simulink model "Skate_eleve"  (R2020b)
settings: Solver=VariableStepAuto  StartTime=0.0  StopTime=10.0  RelTol=1e-3
libraries: fl_lib x8, nesl_utility x4, ee_lib x2, sdl_lib x2

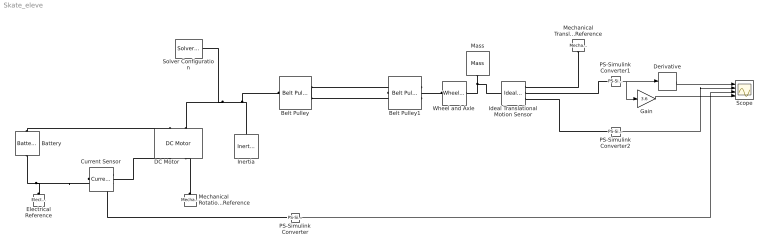
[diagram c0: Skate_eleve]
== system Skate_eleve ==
  Battery : ee_lib/Sources/Battery  Vnom=36 V  prm_dir=1  R1_dis=2 Ohm  R1_ch=2 Ohm  R1=2 Ohm  prm_AH=1  AH=50 hr*A  V1=11.5 V  AH1=25 hr*A  prm_R2=1  R2=2000 Ohm  prm_dyn=1  Rp1=0.005 Ohm  tau1=30 s  Rp2=0.005 Ohm  tau2=30 s  Rp3=0.005 Ohm  tau3=30 s  Rp4=0.005 Ohm  tau4=30 s  Rp5=0.005 Ohm  tau5=30 s  prm_fade=1  N_fade=100  AH_fade=45 hr*A  R1_fade=2.02 Ohm  R1_ch_fade=2.02 Ohm  V1_fade=10.35 V  i_specify=off  i_priority=None  i=0 A  i_nominal_specify=off  i_nominal_unit=A  i_nominal_value=1  v_specify=off  v_priority=None  v=0 V  v_nominal_specify=off  v_nominal_unit=V  v_nominal_value=1  charge_specify=off  charge_priority=High  charge=50 hr*A  charge_nominal_specify=off  charge_nominal_unit=hr*A  charge_nominal_value=1  num_cycles_specify=off  num_cycles_priority=High  num_cycles=0  num_cycles_nominal_specify=off  num_cycles_nominal_unit=1  num_cycles_nominal_value=1  thermal_mass=30000 J/K  Tmeas=298.15 K  Vnom_T2=12 V  R1_T2=2.2 Ohm  R1_T2_dis=2.2 Ohm  R1_T2_ch=2.2 Ohm  V1_T2=11.4 V  R2_T2=2200 Ohm  Rp1_T2=0.005 Ohm  tau1_T2=30 s  Rp2_T2=0.005 Ohm  tau2_T2=30 s  Rp3_T2=0.005 Ohm  tau3_T2=30 s  Rp4_T2=0.005 Ohm  tau4_T2=30 s  Rp5_T2=0.005 Ohm  tau5_T2=30 s  Tmeas2=273.15 K  temperature_specify=off  temperature_priority=High  temperature=298.15 K  temperature_nominal_specify=off  temperature_nominal_unit=K  temperature_nominal_value=1
  Belt Pulley : sdl_lib/Couplings & Drives/Belt Pulley  belt_type=sdl.enum.belt_type.ideal  pulley_moveable=simscape.enum.onoff.off  sheave_ang=30 deg  num_belts=1  model_f_c=sdl.enum.model_centrifugal.off  linear_density=0.6 kg/m  belt_direction=sdl.enum.belt_direction.opposite  breakable=sdl.enum.max_tension.off  F_max=1e5 N  check_tension=sdl.enum.tension_check.off  r_pulley=.15 m  b_pulley=0.001 N*m/(rad/s)  model_inertia=sdl.enum.model_inertia.off  pulley_mass=0.01 kg  initial_vel=0 m/s  pulley_inertia=0.01 kg*m^2  initial_velocity=0 rad/s  mu=0.5  phi_wrap=180 deg  v_thr=0.001 m/s
  Belt Pulley1 : sdl_lib/Couplings & Drives/Belt Pulley  belt_type=sdl.enum.belt_type.ideal  pulley_moveable=simscape.enum.onoff.off  sheave_ang=30 deg  num_belts=1  model_f_c=sdl.enum.model_centrifugal.off  linear_density=0.6 kg/m  belt_direction=sdl.enum.belt_direction.opposite  breakable=sdl.enum.max_tension.off  F_max=1e5 N  check_tension=sdl.enum.tension_check.off  r_pulley=.6 m  b_pulley=0.001 N*m/(rad/s)  model_inertia=sdl.enum.model_inertia.off  pulley_mass=0.01 kg  initial_vel=0 m/s  pulley_inertia=0.01 kg*m^2  initial_velocity=0 rad/s  mu=0.5  phi_wrap=180 deg  v_thr=0.001 m/s
  Current Sensor : fl_lib/Electrical/Electrical Sensors/Current Sensor
  DC Motor : ee_lib/Electromechanical/Brushed Motors/DC Motor  field_option=ee.enum.field_option.pm  Rf=100 Ohm  Lf=1 H  Laf=0.15 H  If0=0 A  parameterization=ee.enum.dcparam_option.circuit_param  Ra=3.9 Ohm  La=12e-6 H  emf_or_torque=ee.enum.emf_or_torque.kv  Kv=0.072e-3 V/rpm  Ki=6.876e-4 N*m/A  T_stall=0.24e-3 N*m  w_max=19100 rpm  w_rated=15000 rpm  P_rated=0.08 W  V_rated=1.5 V  J=0.01 g*cm^2  lam_param=ee.enum.lam_param.damping  lam=0 N*m/(rad/s)  i_noload=0 A  V_i_noload=1.5 V  speed0=0 rpm  enable_fault_armature=ee.enum.faults.faultEnable.no  rev_faulted=1 / 3  G_faulted_armature=1e-5 S  fault_trigger_armature=ee.enum.faults.faultTrigger.temporal  t_fault_armature=1 s  max_permissible_current_armature=inf A  t_fail_on_current_armature=1 s  enable_fault_field=ee.enum.faults.faultEnable.no  G_faulted_field=1e-5 S  fault_trigger_field=ee.enum.faults.faultTrigger.temporal  t_fault_field=1 s  max_permissible_current_field=inf A  t_fail_on_current_field=1 s  fault_action=ee.enum.faults.faultAction.none  alpha=3.93e-3 1/K  Tmeas=25 degC  thermal_mass=100 J/K  initial_temperature=25 degC
  Derivative : Derivative
  Electrical Reference : fl_lib/Electrical/Electrical Elements/Electrical Reference
  Gain : Gain  Gain=3.6
  Ideal Translational Motion Sensor : fl_lib/Mechanical/Mechanical Sensors/Ideal Translational Motion Sensor  offset=0 m
  Inertia : fl_lib/Mechanical/Rotational Elements/Inertia  inertia=0.01 kg*m^2  num_ports=foundation.enum.numPorts2.one  w_specify=off  w_priority=High  w=0 rad/s  w_nominal_specify=off  w_nominal_unit=rad/s  w_nominal_value=1  t_specify=off  t_priority=None  t=0 N*m  t_nominal_specify=off  t_nominal_unit=N*m  t_nominal_value=1
  Mass : fl_lib/Mechanical/Translational Elements/Mass  mass=60 kg  num_ports=foundation.enum.numPorts2.one  v_specify=off  v_priority=High  v=0 m/s  v_nominal_specify=off  v_nominal_unit=m/s  v_nominal_value=1  f_specify=off  f_priority=None  f=0 N  f_nominal_specify=off  f_nominal_unit=N  f_nominal_value=1
  Mechanical Rotational Reference : fl_lib/Mechanical/Rotational Elements/Mechanical Rotational Reference
  Mechanical Translational Reference : fl_lib/Mechanical/Translational Elements/Mechanical Translational Reference
  PS-Simulink Converter : nesl_utility/PS-Simulink Converter  PhysicalDomain=network_engine_domain  SubClassName=ps_output  LeftPortType=input  RightPortType=output  PseudoPeriodic=off  Frequencies=[]  Unit=inherit  AffineConversion=off
  PS-Simulink Converter1 : nesl_utility/PS-Simulink Converter  PhysicalDomain=network_engine_domain  SubClassName=ps_output  LeftPortType=input  RightPortType=output  PseudoPeriodic=off  Frequencies=[]  Unit=inherit  AffineConversion=off
  PS-Simulink Converter2 : nesl_utility/PS-Simulink Converter  PhysicalDomain=network_engine_domain  SubClassName=ps_output  LeftPortType=input  RightPortType=output  PseudoPeriodic=off  Frequencies=[]  Unit=inherit  AffineConversion=off
  Scope : Scope  NumInputPorts=4
  Solver Configuration : nesl_utility/Solver Configuration  PhysicalDomain=network_engine_domain  SubClassName=solver  LeftPortType=input  RightPortType=generic  Tones=[]  Harmonics=[]  SimulateNoise=off  Profile=off  UseLocalSampling=off  EnableSwitchedLinearOptims=on  FrequencyDomain=off  UseCCode=off  RelTol=0.001  AbsTol=1e-06  MinStep=1e-09  ToWorkspace=off  RevertToSquareIcSolve=off  NumHomotopyIterations=100  PhasorMode=off  PhasorModeNumHarmonics=1  DoDC=off  ResidualTolerance=1e-09  UseLocalSolver=off  LocalSolverChoice=NE_BACKWARD_EULER_ADVANCER  LocalSolverSampleTime=0.001  DoFixedCost=off  MaxNonlinIter=3  MaxModeIter=2  ComputeImpulses=off  ImpulseIterations=2  LinearAlgebra=auto  EquationFormulation=NE_TIME_EF  DelaysMemoryBudget=1024  AutomaticFiltering=on  FilteringTimeConstant=0.001  PartitionStorageMethod=AS_NEEDED  PartitionMemoryBudget=1024  PartitionMethod=ROBUST
  Wheel and Axle : fl_lib/Mechanical/Mechanisms/Wheel and Axle  R=0.05 m  or=1  t_specify=off  t_priority=None  t=0 N*m  t_nominal_specify=off  t_nominal_unit=N*m  t_nominal_value=1  f_specify=off  f_priority=None  f=0 N  f_nominal_specify=off  f_nominal_unit=N  f_nominal_value=1
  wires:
  PS-Simulink Converter1/1 -> Gain/1, Derivative/1
  Derivative/1 -> Scope/1
  PS-Simulink Converter2/1 -> Scope/2
  PS-Simulink Converter/1 -> Scope/3
  Gain/1 -> Scope/4
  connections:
  Belt Pulley/RConn1 -- Belt Pulley1/RConn2
  Belt Pulley/RConn2 -- Belt Pulley1/RConn1
  DC Motor/LConn2 -- Solver Configuration/RConn1 -- Inertia/LConn1 -- Belt Pulley/LConn1
  Battery/LConn1 -- DC Motor/LConn1
  Electrical Reference/LConn1 -- Current Sensor/RConn2 -- Battery/RConn1
  Wheel and Axle/LConn1 -- Belt Pulley1/LConn1
  Mechanical Rotational Reference/LConn1 -- DC Motor/RConn2
  Mass/LConn1 -- Ideal Translational Motion Sensor/LConn1 -- Wheel and Axle/RConn1
  Current Sensor/RConn1 -- PS-Simulink Converter/LConn1
  Current Sensor/LConn1 -- DC Motor/RConn1
  Mechanical Translational Reference/LConn1 -- Ideal Translational Motion Sensor/RConn1
  PS-Simulink Converter1/LConn1 -- Ideal Translational Motion Sensor/RConn2
  Ideal Translational Motion Sensor/RConn3 -- PS-Simulink Converter2/LConn1
